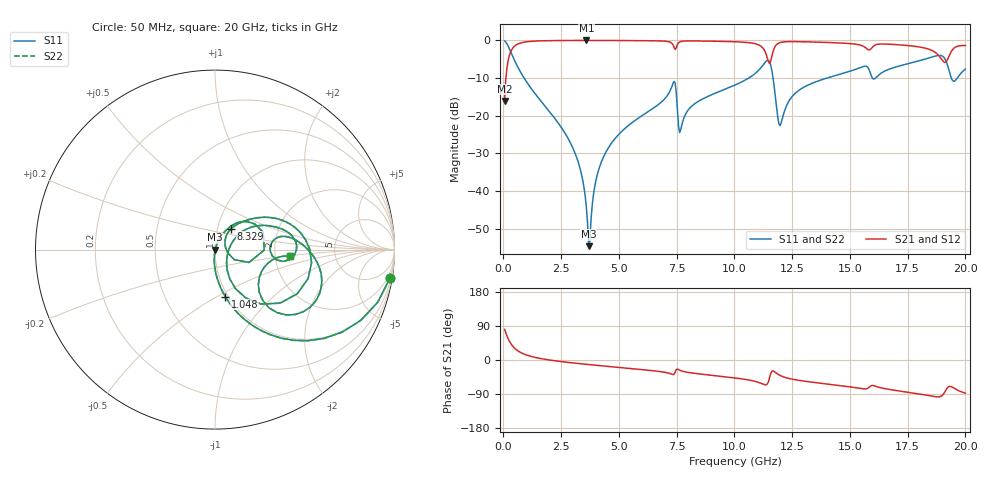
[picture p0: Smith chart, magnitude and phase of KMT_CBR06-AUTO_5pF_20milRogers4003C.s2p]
! Data measured by Modelithics Inc. support@modelithics.com 813-866-6335
! KEMET CBR06-AUTO 5pF, Pad Width= 0.851mm, Pad Length= 0.64mm, Pad Gap= 0.62mm, 20mil Rogers 4003C substrate Data, January 2022
# hz S ma R 50
! 2 Port Network Data from SP1.SP block
! freq  magS11  angS11  magS21  angS21  magS12  angS12  magS22  angS22
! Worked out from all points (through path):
!   401 points, 50 MHz to 20 GHz, reference 50 ohm
!   highest |S21| = -0.01 dB at 3.591 GHz (marker M1); lowest = -16.1 dB at 50 MHz (marker M2)
!   group delay of S21, straight-line fit = 15.2 ps
!   lowest |S11| = -54.6 dB at 3.691 GHz (marker M3), VSWR 1.00, Z = 50.1 - j0.127 ohm
!   |S11| at or under -10 dB: 894 MHz to 10.62 GHz (9.725 GHz wide, 169 % of centre); 11.67 GHz to 14 GHz (2.332 GHz wide, 18.2 % of centre); 19.39 GHz to 19.65 GHz (252.3 MHz wide, 1.29 % of centre)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
!   |S22| runs from -54.6 to -0.1 dB; largest |S21 - S12| = 0
!   S11 on the Smith chart (normalised r, x): 50 MHz: 1, -12; 1.048 GHz: 0.97, -0.55; 8.329 GHz: 1.16, +0.28; 20 GHz: 2.41, -0.22
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5e7  0.9876 -9.2  0.1564 80.8  0.1564 80.8  0.9876 -9.2
3.4925e8  0.6672 -49.2  0.7442 40.7  0.7442 40.7  0.6672 -49.2
1.0475e9  0.268 -77.7  0.9624 12.1  0.9624 12.1  0.268 -77.7
2.74325e9  0.05349 -94.4  0.9971 -5.9  0.9971 -5.9  0.05349 -94.4
3.391625e9  0.01603 -94.7  0.9982 -10.2  0.9982 -10.2  0.01603 -94.7
3.591125e9  0.006047 -86.4  0.9983 -11.4  0.9983 -11.4  0.006047 -86.4
3.690875e9  0.001856 -43.2  0.9983 -12.0  0.9983 -12.0  0.001856 -43.2
4.04e9  0.01546 69.7  0.9981 -14.1  0.9981 -14.1  0.01546 69.7
4.488875e9  0.03521 70.4  0.9975 -16.7  0.9975 -16.7  0.03521 70.4
6.73325e9  0.1429 57.9  0.9846 -30.2  0.9846 -30.2  0.1429 57.9
7.381625e9  0.2852 19.6  0.8175 -38.0  0.8175 -38.0  0.2852 19.6
7.680875e9  0.06613 32.8  0.9661 -28.3  0.9661 -28.3  0.06613 32.8
8.32925e9  0.1478 52.2  0.983 -35.6  0.983 -35.6  0.1478 52.2
1.0025e10  0.2557 41.2  0.9595 -47.3  0.9595 -47.3  0.2557 41.2
1.112225e10  0.4249 21.3  0.8486 -60.8  0.8486 -60.8  0.4249 21.3
1.147138e10  0.5433 -17.3  0.5214 -57.6  0.5214 -57.6  0.5433 -17.3
1.197012e10  0.07383 -12.2  0.934 -40.6  0.934 -40.6  0.07383 -12.2
1.336662e10  0.27 29.4  0.953 -58.6  0.953 -58.6  0.27 29.4
1.670825e10  0.4159 9.7  0.8903 -77.8  0.8903 -77.8  0.4159 9.7
1.910225e10  0.5761 -38.8  0.51 -85.0  0.51 -85.0  0.5761 -38.8
1.950125e10  0.2865 -25.5  0.7862 -74.0  0.7862 -74.0  0.2865 -25.5
2e10  0.4171 -5.1  0.8551 -87.6  0.8551 -87.6  0.4171 -5.1
